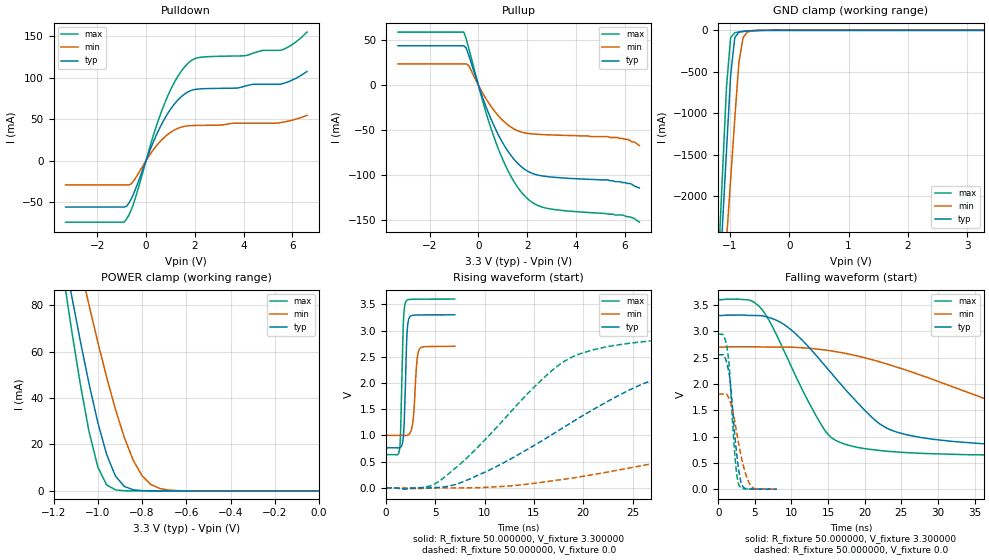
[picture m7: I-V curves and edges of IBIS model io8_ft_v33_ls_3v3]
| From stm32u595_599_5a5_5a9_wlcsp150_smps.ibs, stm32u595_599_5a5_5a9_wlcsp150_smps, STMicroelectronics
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|   Model io8_ft_v33_ls_3v3
[Model]  io8_ft_v33_ls_3v3
Model_type I/O
Polarity   Non-Inverting
Enable   Active-Low
Vinl =   0.990000V
Vinh =   2.310000V
Vmeas =  1.650000V
Cref =   50.000000pF
Rref =   100.000000M
Vref =   0.0V
C_comp   3.252200pF   3.221000pF   3.293600pF
[Temperature Range]   25.000000   0.140000k   -40.000000
[Pullup Reference]   3.300000V   2.700000V   3.600000V
[Pulldown Reference]   0.0V   0.0V   0.0V
[POWER Clamp Reference]   3.300000V   2.700000V   3.600000V
[GND Clamp Reference]   0.0V   0.0V   0.0V
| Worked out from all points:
|   slope of the pulldown table from 0 to 0.495 V, typ, clamps not added: 14 ohm
|   slope of the pullup table from 0 to 0.495 V, typ, clamps not added: 13.7 ohm
|   GND clamp passes 1 mA (typ) near -0.51 V on its own axis
|   POWER clamp passes 1 mA (typ) near -0.85 V on its own axis
|   rising waveform, R_fixture 50.000000, V_fixture 3.300000: 20-80 % time 245ps typ, 337ps min, 229ps max; typ from 0.764 V to 3.3 V
|   rising waveform, R_fixture 50.000000, V_fixture 0.0: 20-80 % time 14.6ns typ, 31.2ns min, 9.34ns max; typ from 0 V to 2.55 V
|   falling waveform, R_fixture 50.000000, V_fixture 3.300000: 20-80 % time 10ns typ, 23.1ns min, 6.37ns max; typ from 3.3 V to 0.764 V
|   falling waveform, R_fixture 50.000000, V_fixture 0.0: 20-80 % time 1.02ns typ, 1.54ns min, 816ps max; typ from 2.55 V to 0 V
[Pulldown]
|Voltage   I(typ)   I(min)   I(max)
-3.3V     -56.06mA   -29.42mA   -74.35mA
-900mV    -56.06mA   -29.42mA   -74.35mA
-700mV    -51.09mA   -29.42mA   -65.48mA
-500mV    -39.32mA   -24.2mA    -50.88mA
300mV     22.62mA    13.13mA    30.43mA
800mV     52.54mA    29.36mA    71.75mA
1.3V      72.91mA    38.82mA    101.4mA
1.8V      84.02mA    42.13mA    119.4mA
2.2V      86.43mA    42.46mA    124.5mA
5.5V      92.01mA    45.75mA    133mA
6.1V      98.6mA     49.6mA     142.1mA
6.6V      107.5mA    54.5mA     155mA
[Pullup]
|Voltage   I(typ)   I(min)   I(max)
-3.3V     43.81mA    23.73mA    58.97mA
-600mV    43.81mA    23.73mA    58.97mA
-500mV    41.28mA    23.73mA    51.53mA
-400mV    33.57mA    21.9mA     41.51mA
300mV     -22.93mA   -14.5mA    -29.27mA
800mV     -54.04mA   -33.36mA   -69.41mA
1.4V      -80.24mA   -47.59mA   -104.2mA
2.1V      -96.56mA   -53.74mA   -127.9mA
3V        -101.9mA   -55.18mA   -137.5mA
5.7V      -107mA     -58mA      -144mA
6.2V      -109mA     -61mA      -146mA
6.6V      -114mA     -67mA      -152mA
[GND_clamp]
|Voltage   I(typ)   I(min)   I(max)
-3.3V     -9.848A    -9.957A    -9.458A
-1.2V     -3.312A    -4.013A    -2.863A
-1.13V    -2.381A    -3.274A    -1.769A
-1.06V    -1.452A    -2.535A    -684.7mA
-990mV    -542.9mA   -1.798A    -88.02mA
-920mV    -87.11mA   -1.064A    -28.44mA
-850mV    -22.1mA    -382.4mA   -19.61mA
-780mV    -11.97mA   -86.98mA   -13.71mA
-710mV    -7.619mA   -22.26mA   -8.745mA
-640mV    -4.493mA   -7.773mA   -4.817mA
-360mV    -31.22uA   -172.6uA   -8.607uA
3.28V     0A         15.66nA    -5.841nA
[POWER_clamp]
|Voltage   I(typ)   I(min)   I(max)
-3.28V    1.355A     1.167A     1.664A
-1.16V    105.7mA    131.6mA    95.69mA
-1.12V    84.97mA    114mA      70.27mA
-1.08V    65.05mA    96.83mA    46.54mA
-1.04V    46.34mA    80.15mA    25.76mA
-1V       29.51mA    64.13mA    10.3mA
-960mV    15.69mA    48.99mA    2.571mA
-920mV    6.373mA    35.1mA     455.6uA
-840mV    490.7uA    13.24mA    11.36uA
-760mV    27.33uA    2.767mA    276.6nA
-640mV    346.6nA    134.1uA    15.48nA
0V        0A         19.91nA    0A
[Ramp]
| variable   typ   min   max
dV/dt_r  1.53252/14.63357n   1.08432/31.20207n   1.76670/9.32647n
dV/dt_f  1.52149/10.01467n   1.01886/23.07548n   1.77964/6.35517n
R_load = 50.000000
[Rising Waveform]
R_fixture= 50.000000
V_fixture= 3.300000
V_fixture_min= 2.700000
V_fixture_max= 3.600000
|time   V(typ)   V(min)   V(max)
0s        764.2mV    1.002V     633.9mV
1.387ns   763.7mV    1.002V     737.1mV
1.499ns   775.3mV    1.002V     1.107V
1.766ns   961.7mV    1.001V     3.111V
2.004ns   2.111V     999.6mV    3.543V
2.13ns    2.894V     1.001V     3.576V
2.298ns   3.203V     1.015V     3.589V
2.733ns   3.291V     1.248V     3.596V
3.391ns   3.297V     2.641V     3.597V
6.979ns   3.3V       2.7V       3.6V
[Rising Waveform]
R_fixture= 50.000000
V_fixture= 0.0
V_fixture_min= 0.0
V_fixture_max= 0.0
|time   V(typ)   V(min)   V(max)
0s        17.53nV    119.4nV    55.53nV
5.506ns   12.1mV     -420.3uV   140.6mV
10.51ns   341.2mV    15.04mV    1.011V
18.52ns   1.214V     176.9mV    2.462V
25.53ns   1.942V     409.4mV    2.776V
29.53ns   2.182V     557mV      2.842V
40.54ns   2.423V     977.4mV    2.913V
55.56ns   2.512V     1.45V      2.938V
76.58ns   2.545V     1.687V     2.944V
249.2ns   2.554V     1.807V     2.944V
[Falling Waveform]
R_fixture= 50.000000
V_fixture= 3.300000
V_fixture_min= 2.700000
V_fixture_max= 3.600000
|time   V(typ)   V(min)   V(max)
0s        3.3V       2.7V       3.6V
4.004ns   3.303V     2.706V     3.6V
6.006ns   3.295V     2.702V     3.409V
10.01ns   3.022V     2.699V     2.321V
15.52ns   2.196V     2.626V     973.5mV
23.02ns   1.159V     2.379V     720.6mV
29.53ns   945mV      2.073V     672.7mV
43.54ns   820.7mV    1.417V     641.9mV
62.56ns   779.7mV    1.15V      635.3mV
249.2ns   764.2mV    1.002V     633.9mV
[Falling Waveform]
R_fixture= 50.000000
V_fixture= 0.0
V_fixture_min= 0.0
V_fixture_max= 0.0
|time   V(typ)   V(min)   V(max)
0s        2.554V     1.807V     2.944V
720.7ps   2.555V     1.807V     2.917V
1.281ns   2.343V     1.778V     2.624V
1.65ns    2.035V     1.662V     2.027V
2.29ns    990.1mV    1.267V     623.3mV
2.531ns   661.6mV    1.071V     287.8mV
2.803ns   360.5mV    859.8mV    89.38mV
3.347ns   50.2mV     496.7mV    11.16mV
4.533ns   1.88mV     50.41mV    2.143mV
7.976ns   17.53nV    119.4nV    55.53nV
